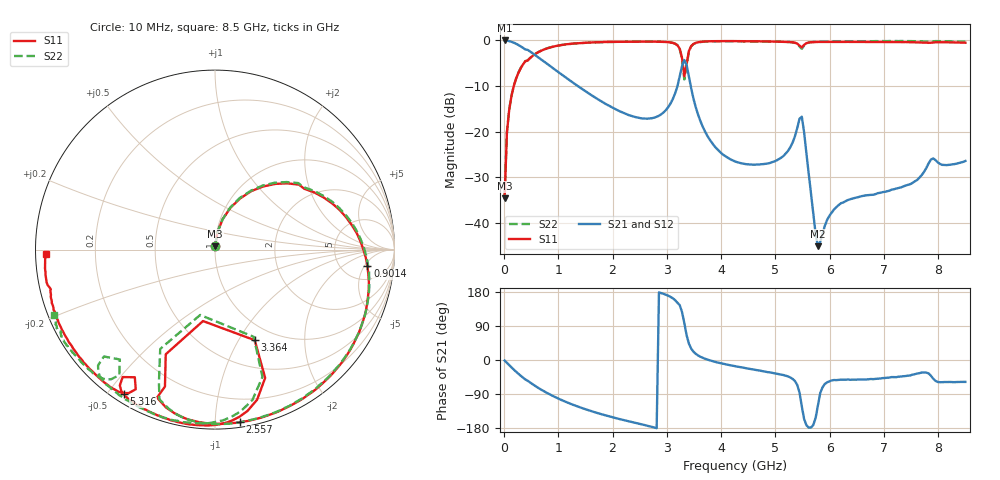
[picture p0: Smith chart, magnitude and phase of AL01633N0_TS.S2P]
!AVX CORPORATION
!PART NUMBER AL01633N0_TS
!DESCRIPTION: AIR CORE INDUCTORS, 33nH, 5 TURNS
!Agilent Technologies,E5071C,MY46102230,A.09.54
!Date: Mon Sep 03 16:33:49 2012
!Data & Calibration Information:
!Freq	S11:SOLT2(ON)	S21:SOLT2(ON)	S12:SOLT2(ON)	S22:SOLT2(ON)
# Hz S dB R 50
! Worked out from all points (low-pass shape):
!   201 points, 10 MHz to 8.5 GHz, reference 50 ohm
!   highest |S21| = 0.00 dB at 10 MHz (marker M1); lowest = -45.1 dB at 5.783 GHz (marker M2)
!   |S21| within 3 dB of the highest: start of sweep to 548.8 MHz
!   lowest |S11| = -34.6 dB at 10 MHz (marker M3), VSWR 1.04, Z = 50 + j1.87 ohm
!   |S11| at or under -10 dB: start of sweep to 179.1 MHz
!   |S22| runs from -34.3 to -0.1 dB; largest |S21 - S12| = 0.014
!   S11 on the Smith chart (normalised r, x): 10 MHz: 1.00, +0.04; 901.5 MHz: 9, -6; 2.557 GHz: 0.03, -1.15; 3.364 GHz: 0.81, -1.17; 5.316 GHz: 0.03, -0.55; 8.5 GHz: 0.03, -0.01
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1e7  -34.57 89.1  -0.00 -1.5  -0.09 -2.1  -34.31 88.0
5.245e7  -20.19 82.0  -0.05 -7.7  -0.03 -7.7  -20.14 82.1
2.2225e8  -8.34 58.3  -0.73 -31.1  -0.71 -31.1  -8.33 58.7
4.7695e8  -3.89 29.9  -2.40 -59.1  -2.39 -59.2  -3.87 30.8
9.0145e8  -1.37 -6.2  -6.08 -95.1  -6.07 -95.2  -1.36 -5.2
1.4533e9  -0.53 -38.7  -10.76 -127.7  -10.76 -127.7  -0.55 -38.4
2.557e9  -0.25 -81.8  -17.12 -170.5  -17.12 -170.6  -0.25 -82.0
2.85415e9  -0.27 -91.9  -16.50 178.4  -16.50 178.3  -0.26 -91.7
3.1513e9  -0.71 -107.2  -11.60 158.0  -11.61 157.9  -0.70 -106.3
3.27865e9  -3.82 -115.2  -5.66 126.9  -5.65 126.9  -3.98 -118.9
3.3211e9  -7.88 -99.5  -4.29 97.7  -4.28 97.7  -8.56 -102.8
3.36355e9  -5.18 -66.3  -5.34 65.2  -5.34 65.2  -5.49 -66.1
3.53335e9  -0.52 -81.8  -14.70 16.1  -14.70 16.1  -0.57 -84.5
4.255e9  -0.15 -100.7  -26.52 -16.3  -26.51 -16.4  -0.21 -108.6
5.31625e9  -0.41 -122.2  -22.39 -49.9  -22.37 -50.0  -0.42 -132.4
5.48605e9  -1.52 -122.1  -16.71 -122.4  -16.72 -122.4  -1.83 -130.9
5.6983e9  -0.36 -125.3  -37.93 -171.2  -37.98 -170.8  -0.35 -132.9
5.7832e9  -0.33 -127.5  -45.09 -119.0  -45.11 -119.8  -0.29 -134.7
6.2077e9  -0.32 -136.8  -35.67 -51.8  -35.87 -51.4  -0.23 -140.5
7.09915e9  -0.34 -154.1  -32.93 -46.5  -32.97 -46.2  -0.13 -148.1
7.9057e9  -0.46 -167.5  -25.85 -49.0  -25.88 -49.1  -0.22 -152.0
8.5e9  -0.50 -178.4  -26.42 -57.8  -26.44 -57.9  -0.29 -158.0
